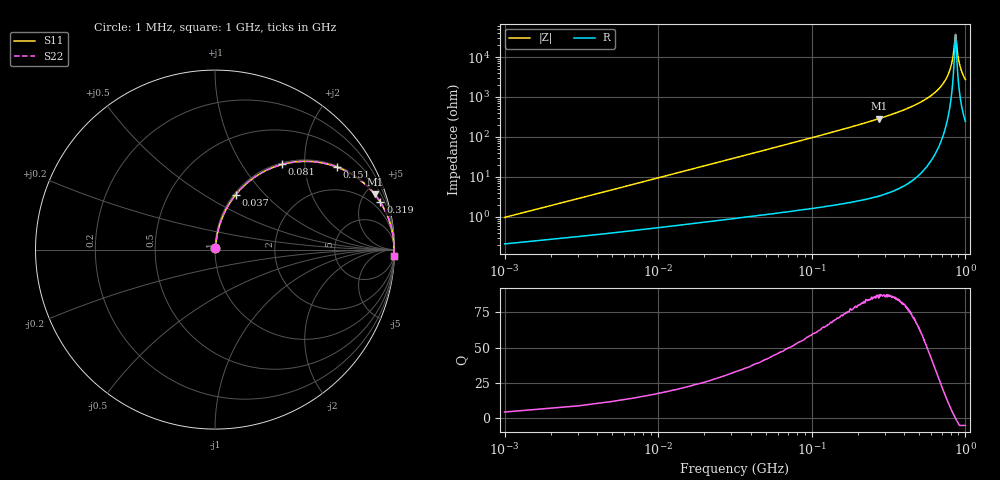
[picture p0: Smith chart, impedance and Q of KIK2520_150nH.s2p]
!version-2
!date-01.2022
!Series
# MHz S RI R 50
!Freq ReS11 ImS11 ReS21 ImS21 ReS12 ImS12 ReS22 ImS22
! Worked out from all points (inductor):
!   501 points, 1 MHz to 1 GHz, reference 50 ohm
!   read as one part in series: L = 150 nH near 5 MHz
!   highest Q = 87.1 at 275 MHz (marker M1), where L = 167 nH
!   self-resonance near 861 MHz
!   S11 on the Smith chart (normalised r, x): 1 MHz: 1.00, +0.02; 37 MHz: 1.02, +0.70; 81 MHz: 1.03, +1.54; 151 MHz: 1.04, +2.94; 319 MHz: 1.08, +6.97; 1 GHz: 6, -54
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1  0.00216 0.00938  0.9978 -0.00938  0.9978 -0.00938  0.00216 0.00938
7  0.00882 0.0651  0.9912 -0.0651  0.9912 -0.0651  0.00882 0.0651
13  0.0205 0.1193  0.9795 -0.1193  0.9795 -0.1193  0.0205 0.1193
23  0.0517 0.2041  0.9483 -0.2041  0.9483 -0.2041  0.0517 0.2041
37  0.1156 0.306  0.8844 -0.306  0.8844 -0.306  0.1156 0.306
81  0.3747 0.4748  0.6253 -0.4748  0.6253 -0.4748  0.3747 0.4748
151  0.6808 0.4592  0.3192 -0.4592  0.3192 -0.4592  0.6808 0.4592
169  0.7302 0.4372  0.2698 -0.4372  0.2698 -0.4372  0.7302 0.4372
275  0.89 0.3072  0.11 -0.3072  0.11 -0.3072  0.89 0.3072
319  0.9213 0.2636  0.0787 -0.2636  0.0787 -0.2636  0.9213 0.2636
335  0.93 0.2493  0.07 -0.2493  0.07 -0.2493  0.93 0.2493
501  0.9786 0.137  0.0214 -0.137  0.0214 -0.137  0.9786 0.137
667  0.9937 0.0634  0.00626 -0.0634  0.00626 -0.0634  0.9937 0.0634
775  0.9969 0.0262  0.00313 -0.0262  0.00313 -0.0262  0.9969 0.0262
811  0.9972 0.0151  0.00277 -0.0151  0.00277 -0.0151  0.9972 0.0151
835  0.9973 0.00797  0.00268 -0.00797  0.00268 -0.00797  0.9973 0.00797
857  0.9973 0.00161  0.00269 -0.00161  0.00269 -0.00161  0.9973 0.00161
863  0.9973 -0.0001  0.00271 0.0001  0.00271 0.0001  0.9973 -0.0001
889  0.9971 -0.00736  0.00286 0.00736  0.00286 0.00736  0.9971 -0.00736
913  0.9969 -0.0139  0.00309 0.0139  0.00309 0.0139  0.9969 -0.0139
949  0.9964 -0.0233  0.00359 0.0233  0.00359 0.0233  0.9964 -0.0233
1000  0.9954 -0.0362  0.00459 0.0362  0.00459 0.0362  0.9954 -0.0362
